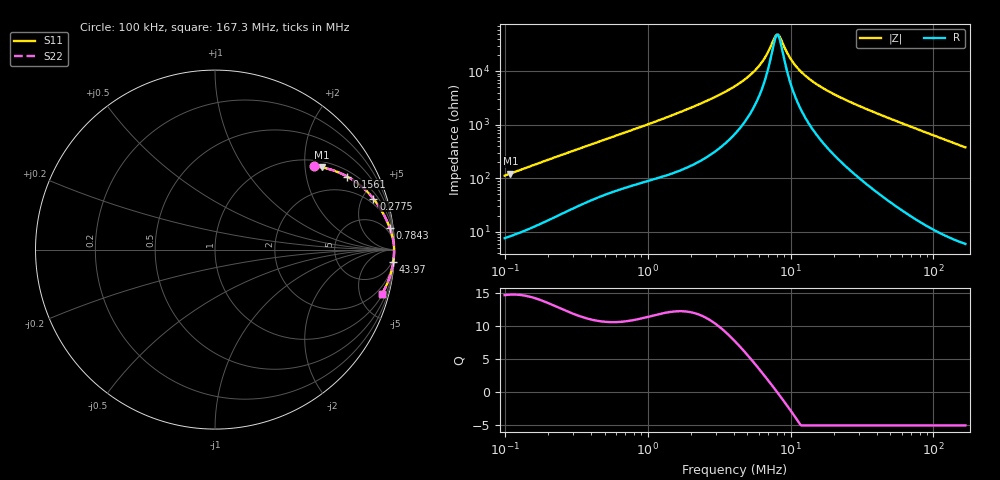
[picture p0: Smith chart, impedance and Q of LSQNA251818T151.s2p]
! LSQNA251818T151  S-PARAMETER MODEL  ( General Type )
! Model Generated by TAIYO YUDEN Corporation (http://www.ty-top.com)
! Version 2.0
! TAIYO YUDEN Control No. 100810NF25SB-FKC
! Copyright(c) 2007 TAIYO YUDEN CO.,LTD. All Rights Reserved.
! Product Description (link to TY-COMPAS)
! https://ds.yuden.co.jp/TYCOMPAS/or/detail?pn=LSQNA251818T151K&u=M
! Products Name : Inductors
! Characteristics :
!  Inductance : 150 uH , SRF(min) : 7.0 MHz , DC Resistance(max) : 4.16 Ohm
!  Rated Current : Saturation :55 mA , Temp Rise : 210 mA (40 degC)
!  Case Size : 2.5 x 1.8 / 0.098 x 0.071 [mm/inch] , Thickness : 1.8 / 0.071 [mm/inch]
!  (Conditions: Temperature = 25 degC , DC Bias Current/Voltage = 0A / 0V)
! External Node Assignments :
!  1  o---GGG---o  2
! GND o---------o GND
! Frequency Range : 0.1MHz  -  167.251077MHz  [ 402 STEP ]
# MHz S RI R 50
! Freq[MHz].  S11 Real  S11 Imag  S21 Real  S21 Imag  S12 Real  S12 Imag  S22 Real  S22 Imag
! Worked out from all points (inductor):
!   401 points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, 100 kHz to 167.3 MHz, reference 50 ohm
!   read as one part in series: L = 177 uH near 103.8 kHz
!   highest Q = 14.8 at 109.7 kHz (marker M1), where L = 178 uH
!   self-resonance near 7.976 MHz
!   S11 on the Smith chart (normalised r, x): 100 kHz: 1.15, +2.24; 156.1 kHz: 1.24, +3.46; 277.5 kHz: 1.49, +6.02; 784.3 kHz: 2, +16; 43.97 MHz: 2, -30; 167.3 MHz: 1.12, -7.57
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0.1  0.554 0.4642  0.446 -0.4642  0.446 -0.4642  0.554 0.4642
0.109722  0.5956 0.4581  0.4044 -0.4581  0.4044 -0.4581  0.5956 0.4581
0.1561  0.7365 0.4071  0.2635 -0.4071  0.2635 -0.4071  0.7365 0.4071
0.277468  0.8825 0.2836  0.1175 -0.2836  0.1175 -0.2836  0.8825 0.2836
0.346668  0.9147 0.2389  0.0853 -0.2389  0.0853 -0.2389  0.9147 0.2389
0.784305  0.974 0.1197  0.026 -0.1197  0.026 -0.1197  0.974 0.1197
1.20179  0.9866 0.0804  0.0134 -0.0804  0.0134 -0.0804  0.9866 0.0804
2.571721  0.9955 0.0357  0.00446 -0.0357  0.00446 -0.0357  0.9955 0.0357
4.166227  0.9973 0.0181  0.00274 -0.0181  0.00274 -0.0181  0.9973 0.0181
5.109584  0.9976 0.0121  0.00239 -0.0121  0.00239 -0.0121  0.9976 0.0121
6.038253  0.9978 0.00755  0.00221 -0.00755  0.00221 -0.00755  0.9978 0.00755
6.749349  0.9979 0.00464  0.00213 -0.00464  0.00213 -0.00464  0.9979 0.00464
7.685477  0.9979 0.00131  0.00206 -0.00131  0.00206 -0.00131  0.9979 0.00131
8.125425  0.998 -0.000113  0.00205 0.000113  0.00205 0.000113  0.998 -0.000113
8.432628  0.998 -0.00106  0.00204 0.00106  0.00204 0.00106  0.998 -0.00106
9.602225  0.998 -0.00439  0.00203 0.00439  0.00203 0.00439  0.998 -0.00439
10.53571  0.998 -0.00682  0.00204 0.00682  0.00204 0.00682  0.998 -0.00682
14.17747  0.9978 -0.0151  0.0022 0.0151  0.0022 0.0151  0.9978 -0.0151
21.72413  0.9972 -0.0295  0.00284 0.0295  0.00284 0.0295  0.9972 -0.0295
43.97061  0.9935 -0.0667  0.00654 0.0667  0.00654 0.0667  0.9935 -0.0667
49.14881  0.9922 -0.075  0.00777 0.075  0.00777 0.075  0.9922 -0.075
167.2511  0.9314 -0.245  0.0686 0.245  0.0686 0.245  0.9314 -0.245
